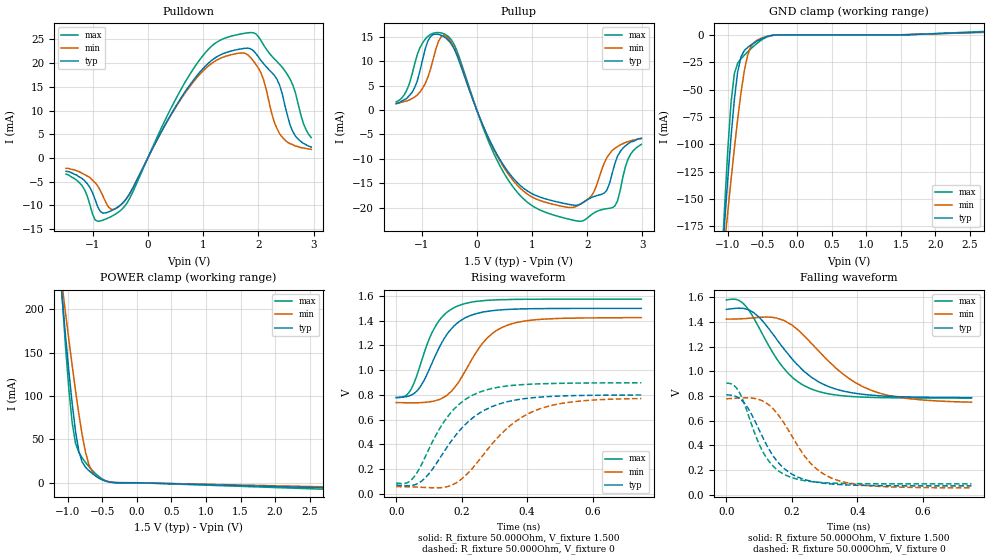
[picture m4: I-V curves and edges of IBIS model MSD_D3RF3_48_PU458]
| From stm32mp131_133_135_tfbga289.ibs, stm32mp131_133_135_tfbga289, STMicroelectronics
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[Model] MSD_D3RF3_48_PU458
Model_type   I/O
C_comp 2.387pF   2.305pF   2.510pF
Vinh = 925.000mV
Vinl = 575.000mV
Vmeas = 750.000mV
Vref = 750.000mV
[Model Spec]
Vinh   925.000mV   888.000mV   963.000mV
Vinl   575.000mV   538.000mV   613.000mV
Vmeas   750.000mV   713.000mV   788.000mV
Vref   750.000mV   713.000mV   788.000mV
[Temperature Range]   25.000   125.000   -40.000
[Voltage Range]   1.500V   1.425V   1.575V
[GND Clamp Reference]   0.00V   0.00V   0.00V
[Pulldown Reference]   0.00V   0.00V   0.00V
[POWER Clamp Reference]   1.500V   1.425V   1.575V
[Pullup Reference]   1.500V   1.425V   1.575V
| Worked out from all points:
|   slope of the pulldown table from 0 to 0.225 V, typ, clamps not added: 44.1 ohm
|   slope of the pullup table from 0 to 0.225 V, typ, clamps not added: 37.5 ohm
|   GND clamp passes 1 mA (typ) near -0.40 V on its own axis
|   POWER clamp passes 1 mA (typ) near -0.41 V on its own axis
|   rising waveform, R_fixture 50.000Ohm, V_fixture 1.500: 20-80 % time 89.7ps typ, 107ps min, 75.1ps max; typ from 0.779 V to 1.5 V
|   rising waveform, R_fixture 50.000Ohm, V_fixture 0: 20-80 % time 139ps typ, 159ps min, 118ps max; typ from 0.069 V to 0.798 V
|   falling waveform, R_fixture 50.000Ohm, V_fixture 1.500: 20-80 % time 147ps typ, 173ps min, 119ps max; typ from 1.5 V to 0.788 V
|   falling waveform, R_fixture 50.000Ohm, V_fixture 0: 20-80 % time 99.3ps typ, 117ps min, 81.9ps max; typ from 0.81 V to 0.072 V
[GND Clamp]
-1.48V    -594.4mA   -480.1mA   -764mA
-1.098V   -218.6mA   -223.6mA   -220.7mA
-1.05V    -174.5mA   -192.7mA   -160.1mA
-1.002V   -132.2mA   -162.2mA   -105.7mA
-954.6mV  -93.12mA   -132.5mA   -61.92mA
-906.8mV  -59.28mA   -104.1mA   -35.5mA
-859.1mV  -34.03mA   -77.35mA   -25.95mA
-811.4mV  -20.11mA   -53.24mA   -21.91mA
-715.9mV  -11.56mA   -18.86mA   -15.62mA
-572.7mV  -5.498mA   -4.705mA   -7.443mA
-286.4mV  -67.01uA   -116.4uA   -54.62uA
2.959V    3.204mA    2.733mA    3.866mA
[Power Clamp]
-1.459V   578.3mA    479.7mA    723.8mA
-1.077V   211.4mA    225.9mA    210.8mA
-1.03V    168.5mA    195mA      156.1mA
-981.8mV  127.9mA    164.6mA    107.2mA
-934.1mV  90.82mA    134.9mA    68.67mA
-886.4mV  59.31mA    106.4mA    45.54mA
-838.6mV  36.44mA    79.64mA    34.94mA
-743.2mV  18.07mA    35.72mA    23.56mA
-647.7mV  10.89mA    12.97mA    14.52mA
-552.3mV  5.57mA     5.518mA    7.336mA
-313.6mV  106.2uA    243.6uA    119.9uA
2.98V     -6.459mA   -5.197mA   -8.237mA
[Pulldown]
-1.48V    -2.8mA     -2.2mA     -3.4mA
-1.193V   -4.3mA     -3.2mA     -5.8mA
-954.6mV  -8.75mA    -5.2mA     -13.05mA
-811.4mV  -11.64mA   -8.06mA    -13.11mA
-525mV    -10.19mA   -10.28mA   -11.38mA
906.8mV   17.61mA    17.2mA     20.18mA
1.241V    21.28mA    20.6mA     24.36mA
1.766V    23.14mA    22.05mA    26.32mA
2.052V    20.52mA    17.85mA    24.7mA
2.386V    15.36mA    5.1mA      19.75mA
2.625V    5.6mA      2.8mA      15.4mA
2.959V    2.3mA      1.8mA      4.3mA
[Pullup]
-1.459V   1.3mA      1.357mA    1.686mA
-1.125V   4.6mA      2.671mA    9.443mA
-934.1mV  12.53mA    5.429mA    14.53mA
-695.5mV  15.51mA    14.06mA    15.89mA
-552.3mV  14.7mA     15.08mA    15.38mA
640.9mV   -13.72mA   -14.18mA   -15.51mA
1.834V    -19.47mA   -19.54mA   -22.76mA
2.12V     -17.72mA   -16.78mA   -21.08mA
2.311V    -16.98mA   -10.74mA   -20.29mA
2.502V    -10.9mA    -7.829mA   -19.63mA
2.741V    -6.9mA     -6.443mA   -9.986mA
2.98V     -5.8mA     -5.8mA     -7.029mA
[Ramp]
R_load=50.000Ohm
dV/dt_r   432.363mV/115.500ps  419.793mV/134.000ps  480.240mV/96.500ps
dV/dt_f   432.363mV/123.500ps  419.763mV/148.000ps  480.240mV/101.000ps
[Rising waveform]
R_fixture=50.000Ohm
V_fixture=1.500
V_fixture_min=1.425
V_fixture_max=1.575
0s        779.3mV    737.5mV    777mV
39ps      790.4mV    735.5mV    818.4mV
69ps      848.9mV    736.1mV    1.004V
123ps     1.137V     754.9mV    1.369V
154ps     1.286V     794.2mV    1.466V
192ps     1.392V     908.1mV    1.524V
268ps     1.472V     1.23V      1.563V
337ps     1.491V     1.361V     1.571V
444ps     1.498V     1.412V     1.574V
749ps     1.5V       1.425V     1.575V
[Rising waveform]
R_fixture=50.000Ohm
V_fixture=0
0s        68.74mV    56.17mV    84.82mV
46ps      64.96mV    54.05mV    109.7mV
85ps      118.1mV    50.03mV    276.5mV
161ps     398.1mV    59.57mV    636.1mV
199ps     526.3mV    116.1mV    738.4mV
253ps     649.8mV    270.1mV    819.8mV
345ps     747.5mV    543.2mV    873.5mV
437ps     781mV      684.6mV    888.8mV
544ps     793.5mV    744.5mV    894.6mV
749ps     798.5mV    769.9mV    897.4mV
[Falling waveform]
R_fixture=50.000Ohm
V_fixture=1.500
V_fixture_min=1.425
V_fixture_max=1.575
0s        1.503V     1.424V     1.579V
46ps      1.512V     1.427V     1.563V
85ps      1.473V     1.435V     1.427V
177ps     1.179V     1.412V     1.021V
215ps     1.06V      1.345V     923.2mV
261ps     950.6mV    1.224V     856.3mV
360ps     839.2mV    971.9mV    801.6mV
444ps     807.9mV    845.7mV    789.5mV
552ps     793.7mV    780.9mV    785.3mV
749ps     788.3mV    751mV      783.8mV
[Falling waveform]
R_fixture=50.000Ohm
V_fixture=0
0s        809.5mV    778.6mV    904.9mV
39ps      784.2mV    784.3mV    834.6mV
69ps      690.3mV    785.7mV    633.5mV
115ps     445mV      755mV      332.8mV
154ps     276.2mV    663.8mV    205.6mV
192ps     182mV      513.6mV    147.6mV
261ps     109.5mV    246mV      107mV
345ps     83.33mV    113.4mV    93.33mV
467ps     74.08mV    68.29mV    89.52mV
749ps     71.99mV    56.48mV    88.84mV
